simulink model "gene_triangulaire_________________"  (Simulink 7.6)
settings: Solver=ode15s  StartTime=0.0  StopTime=2  RelTol=1e-3
libraries: fl_lib x8, elec_lib x2, nesl_utility x2

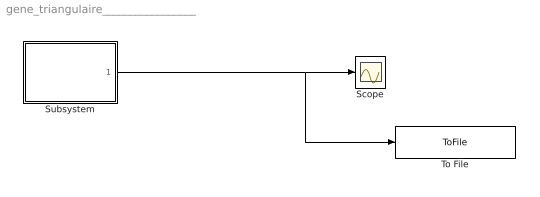
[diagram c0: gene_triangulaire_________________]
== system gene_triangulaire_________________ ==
  Scope : Scope
  Subsystem : Subsystem
  To File : ToFile  Filename=signal_triangle  MatrixName=x
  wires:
  Subsystem/1(tri) -> Scope/1, To File/1

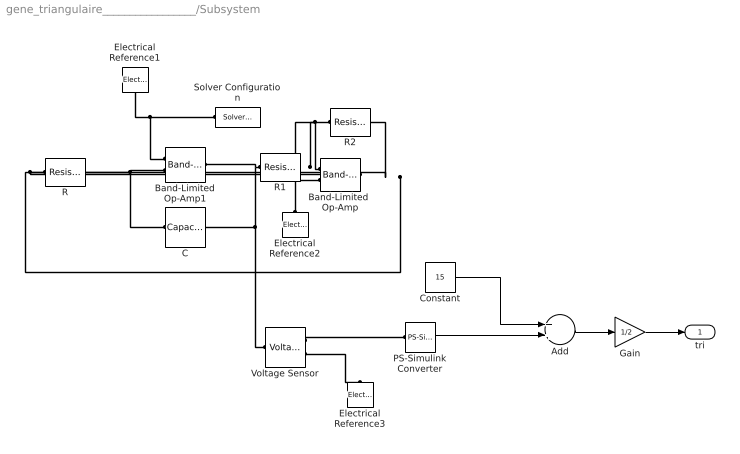
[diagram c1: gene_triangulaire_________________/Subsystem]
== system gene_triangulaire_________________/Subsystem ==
  Add : Sum
  Band-Limited  Op-Amp : elec_lib/Integrated Circuits/Band-Limited Op-Amp  DialogController=NetworkEngine.DynNeDlgSource  SystemSampleTime=-1  A=1000  Rin=1e+06 Ohm  Rout=100 Ohm  Vmin=-15 V  Vmax=15 V  Vdotmax=1000 V/s  f=1e+05 Hz  V0=0 V  LocalVarNames=|power  LocalVarDescs=|Dissipated power (W)  LocalVarLogging=0
  Band-Limited Op-Amp1 : elec_lib/Integrated Circuits/Band-Limited Op-Amp  DialogController=NetworkEngine.DynNeDlgSource  SystemSampleTime=-1  A=1000  Rin=1e+06 Ohm  Rout=100 Ohm  Vmin=-15 V  Vmax=15 V  Vdotmax=1000 V/s  f=1e+05 Hz  V0=0 V  LocalVarNames=|power  LocalVarDescs=|Dissipated power (W)  LocalVarLogging=0
  C : fl_lib/Electrical/Electrical Elements/Capacitor  DialogController=NetworkEngine.DynNeDlgSource  SystemSampleTime=-1  c=1e-6 F  v0=0.1 V  r=1e-6 Ohm  g=0 1/Ohm  i_Log=off  v_Log=off  vc_Log=off  LocalVarNames=|current|voltage|power  LocalVarDescs=|Capacitor current (A)|Voltage across capacitor (V)|Power (W)  LocalVarLogging=[0 0 0]
  Constant : Constant  Value=15
  Electrical Reference1 : fl_lib/Electrical/Electrical Elements/Electrical Reference  DialogController=NetworkEngine.DynNeDlgSource  SystemSampleTime=-1  i_Log=off  LocalVarNames=|i  LocalVarDescs=|i  LocalVarLogging=[]
  Electrical Reference2 : fl_lib/Electrical/Electrical Elements/Electrical Reference  DialogController=NetworkEngine.DynNeDlgSource  SystemSampleTime=-1  i_Log=off  LocalVarNames=|i  LocalVarDescs=|i  LocalVarLogging=[]
  Electrical Reference3 : fl_lib/Electrical/Electrical Elements/Electrical Reference  DialogController=NetworkEngine.DynNeDlgSource  SystemSampleTime=-1  i_Log=off  LocalVarNames=|i  LocalVarDescs=|i  LocalVarLogging=[]
  Gain : Gain  Gain=1/2
  PS-Simulink Converter : nesl_utility/PS-Simulink Converter  DialogController=NetworkEngine.DynNeUtilDlgSource  SystemSampleTime=-1  PhysicalDomain=network_engine_domain  LeftPortType=input  RightPortType=output  SubClassName=ps_output  Unit=1  AffineConversion=off
  R : fl_lib/Electrical/Electrical Elements/Resistor  DialogController=NetworkEngine.DynNeDlgSource  SystemSampleTime=-1  R=100e3 Ohm  i_Log=off  v_Log=off  LocalVarNames=|current|voltage|power  LocalVarDescs=|Resistor current (A)|Voltage across resistor (V)|Power (W)  LocalVarLogging=[0 0 0]
  R1 : fl_lib/Electrical/Electrical Elements/Resistor  DialogController=NetworkEngine.DynNeDlgSource  SystemSampleTime=-1  R=10e3 Ohm  i_Log=off  v_Log=off  LocalVarNames=|current|voltage|power  LocalVarDescs=|Resistor current (A)|Voltage across resistor (V)|Power (W)  LocalVarLogging=[0 0 0]
  R2 : fl_lib/Electrical/Electrical Elements/Resistor  DialogController=NetworkEngine.DynNeDlgSource  SystemSampleTime=-1  R=10e3 Ohm  i_Log=off  v_Log=off  LocalVarNames=|current|voltage|power  LocalVarDescs=|Resistor current (A)|Voltage across resistor (V)|Power (W)  LocalVarLogging=[0 0 0]
  Solver Configuration : nesl_utility/Solver Configuration  DialogController=NetworkEngine.DynNeUtilDlgSource  SystemSampleTime=-1  PhysicalDomain=network_engine_domain  LeftPortType=input  RightPortType=generic  SubClassName=solver  Accelerate=off  Profile=off  ResidualTolerance=1e-9  MaxNonlinIter=12  MaxModeIter=2  DoFixedCost=off  UseLocalSampling=off  DoDC=off  LinearAlgebra=Sparse  LocalSolverSampleTime=.001  LocalSolverChoice=NE_BACKWARD_EULER_ADVANCER  UseLocalSolver=off
  Voltage Sensor : fl_lib/Electrical/Electrical Sensors/Voltage Sensor  DialogController=NetworkEngine.DynNeDlgSource  SystemSampleTime=-1  i1_Log=off  v1_Log=off  LocalVarNames=|i1|v1  LocalVarDescs=|i1|v1  LocalVarLogging=[]
  tri : Outport
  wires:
  PS-Simulink Converter/1 -> Add/2
  Constant/1 -> Add/1
  Add/1 -> Gain/1
  Gain/1 -> tri/1
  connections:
  Voltage Sensor/RConn1 -- PS-Simulink Converter/LConn1
  Voltage Sensor/LConn1 -- Band-Limited Op-Amp1/RConn1 -- R1/LConn1 -- C/RConn1
  C/LConn1 -- Band-Limited Op-Amp1/LConn2 -- R/RConn1
  Solver Configuration/RConn1 -- Band-Limited Op-Amp1/LConn1 -- Electrical Reference1/LConn1
  R/LConn1 -- Band-Limited  Op-Amp/RConn1 -- R2/RConn1
  Electrical Reference2/LConn1 -- Band-Limited  Op-Amp/LConn2
  R2/LConn1 -- Band-Limited  Op-Amp/LConn1 -- R1/RConn1
  Voltage Sensor/RConn2 -- Electrical Reference3/LConn1
